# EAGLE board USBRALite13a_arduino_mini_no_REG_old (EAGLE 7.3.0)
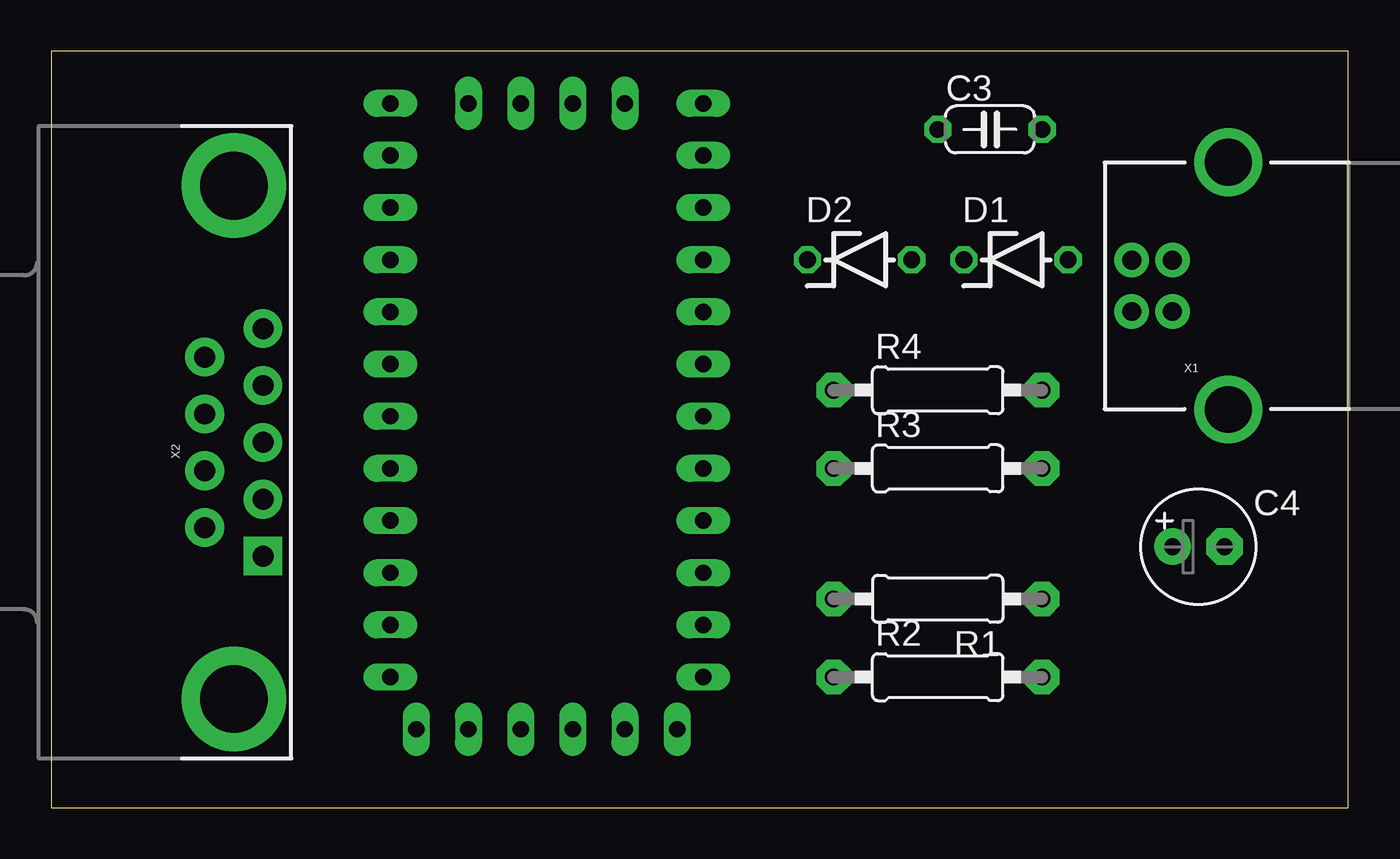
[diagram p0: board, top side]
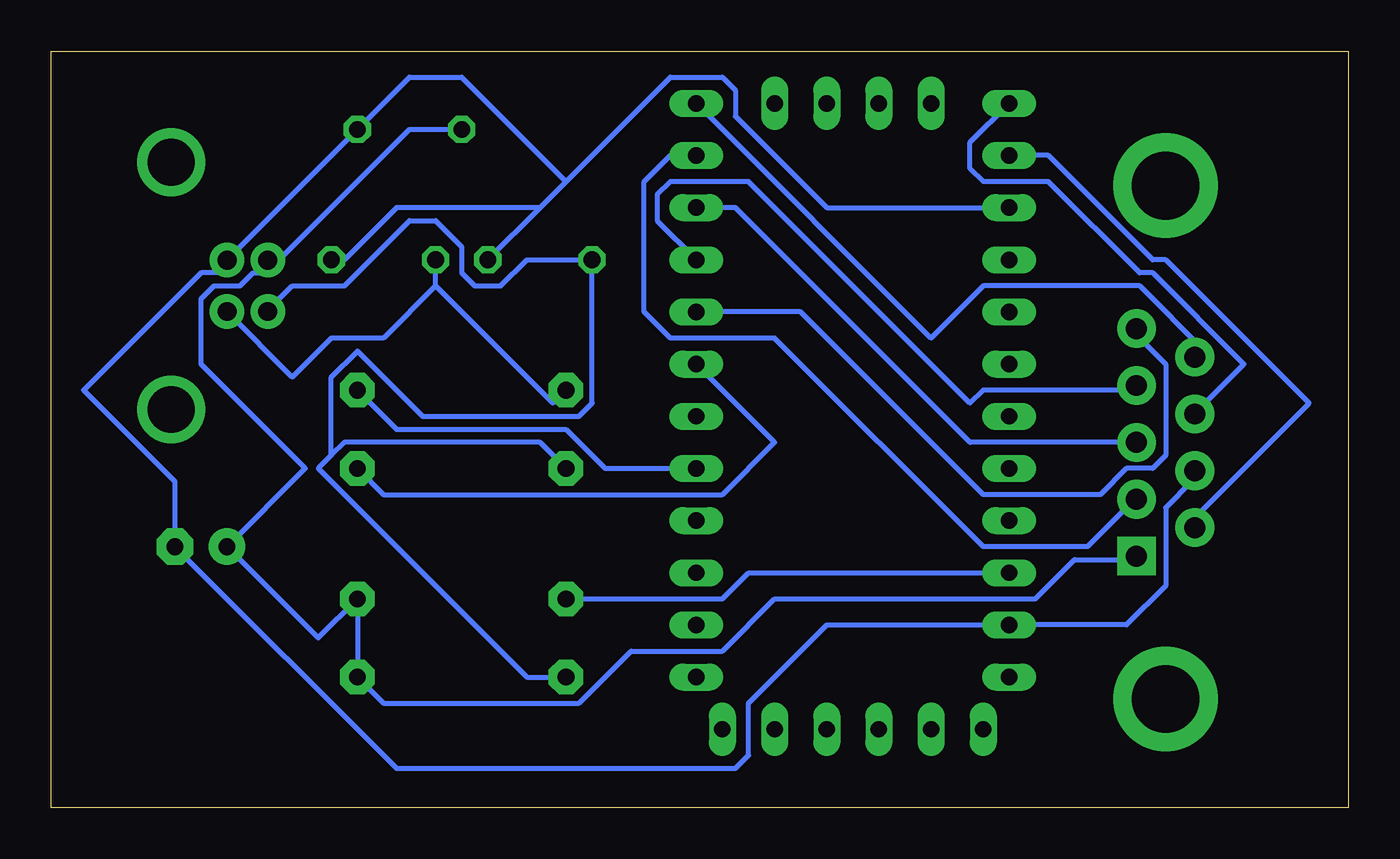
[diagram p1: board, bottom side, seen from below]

Size 63.17 x 36.82 mm. Coordinates in mm from the lower left corner, seen from the top.
Outline: 0,0 63.17,0 63.17,36.82 0,36.82 0,0
Copper layers (1*16): Top 0.035mm / dielectric 1.5mm / Bottom 0.035mm
Design rules "default": minimum track width 10mil, minimum drill 24mil, track to track 8mil, track to pad 8mil, pad to pad 8mil, via to via 8mil, smd to smd 8mil, copper to edge 40mil, drill to drill 8mil, minimum pad ring 10mil, minimum via ring 8mil, stop-mask expansion 4mil, vias tented up to drill 0mil, thermal gap 10mil

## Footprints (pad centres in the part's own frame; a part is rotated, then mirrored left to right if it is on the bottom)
C050-024X044 = drill 0.813 octagon: 1 -2.54,0; 2 2.54,0
E2,5-6 = drill 0.813 pad 1.778: + -1.27,0 | drill 0.813 pad 1.778 octagon: - 1.27,0
ZDIO-5 = drill 0.813 octagon: A 2.54,0; C -2.54,0
0207/10 = drill 0.813 pad 1.676 octagon: 1 -5.08,0; 2 5.08,0
PRO-MINI = drill 0.8 long: A0 8.89,8.89; A1 8.89,11.43; A2 8.89,13.97; A3 8.89,16.51; A4 -2.54,-1.27; A5 0,-1.27; A6 2.54,-1.27; A7 5.08,-1.27; D2 -6.35,16.51; D3 -6.35,13.97; D4 -6.35,11.43; D5 -6.35,8.89; D6 -6.35,6.35; D7 -6.35,3.81; D8 -6.35,1.27; D9 -6.35,-1.27; D10 8.89,-1.27; D11 8.89,1.27; D12 8.89,3.81; D13 8.89,6.35; DTR 7.62,29.21; GND 8.89,24.13; GND1 -6.35,19.05; GND2 -5.08,29.21; GND3 -2.54,29.21; RAW 8.89,26.67; RST 8.89,21.59; RST1 -6.35,21.59; RX1 -6.35,24.13; RX1-1 2.54,29.21; TX0 -6.35,26.67; TX0-1 5.08,29.21; VCC 8.89,19.05; VCC1 0,29.21
USB-B-PTH = drill 0.914 pad 1.676: D+ 0,1.25; D- 1.981,1.25; GND 0,-1.25; VBUS 1.981,-1.25 | drill 2.286: S1 -2.718,-6.02; S2 -2.718,6.02
DB9_MALE = drill 1.016 pad 1.88: 1 5.54,-1.42; 2 2.77,-1.42; 3 0,-1.42; 4 -2.77,-1.42; 6 4.15,1.42; 7 1.38,1.42; 8 -1.38,1.42; 9 -4.15,1.42 | drill 1.016 pad 1.88 square: 5 -5.54,-1.42 | drill 3.302 pad 5.08: G1 -12.5,0; G2 12.5,0

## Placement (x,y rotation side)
C3  0.1uF  [C050-024X044]  45.72,33.02 0 top
C4  4u7  [E2,5-6]  55.88,12.7 0 top
D1  3V6  [ZDIO-5]  46.99,26.67 0 top
D2  3V6  [ZDIO-5]  39.37,26.67 0 top
R1  10K  [0207/10]  43.18,10.16 180 top
R2  1K5  [0207/10]  43.18,6.35 0 top
R3  68R  [0207/10]  43.18,16.51 0 top
R4  68R  [0207/10]  43.18,20.32 0 top
U$1  PRO-MINI  [PRO-MINI]  25.4,33.02 180 top
X1  USBPTH  [USB-B-PTH]  54.61,25.4 180 top
X2  [DB9_MALE]  8.89,17.78 90 top

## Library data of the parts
C3 = rcl
C4 R1-R4 = adafruit
D1 D2 = diode
U$1 = Arduino-clone
X1 X2 = SparkFun

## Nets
D+: R4.2 U$1.D2
D-: R3.2 U$1.D4
GND: C3.2 C4.- D1.A D2.A U$1.D12 U$1.GND X1.GND X2.8
N$1: R1.2 U$1.RST
N$8: D1.C R4.1 X1.D+
N$9: D2.C R2.1 R3.1 X1.D-
PB0: U$1.D8 X2.4
PB1: U$1.D9 X2.6
PB2: U$1.D10 X2.7
PB3: U$1.D11 X2.9
PD5: U$1.D5 X2.1
PD7: U$1.D7 X2.3
PD62: U$1.D6 X2.2
RAW: U$1.RAW
VCC: C3.1 C4.+ R1.1 R2.2 X1.VBUS X2.5

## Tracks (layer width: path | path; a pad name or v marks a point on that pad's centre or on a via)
D+
  Bottom 0.254: U$1.D2 36.2,16.51 38.1,18.41 46.35,18.41 R4.2
D-
  Bottom 0.254: U$1.D4 27.94,17.78 30.48,15.24 46.99,15.24 R3.2
GND
  Bottom 0.254: U$1.D12 25.4,29.21 29.84,33.66 29.84,34.92 30.48,35.56 33.02,35.56 38.1,30.48 | D2.A 39.37,29.21 | 39.37,29.21 38.1,30.48 | D1.A 48.9,26.67 46.35,29.21 39.37,29.21 | X2.8 7.62,15.88 8.89,14.6 8.89,10.79 10.79,8.89 U$1.GND 25.4,8.89 29.21,5.08 29.21,2.54 29.84,1.9 46.35,1.9 C4.- 57.15,15.88 61.59,20.32 55.88,26.03 54.61,26.03 X1.GND 54.61,26.67 C3.2 45.72,35.56 43.18,35.56 38.1,30.48
N$1
  Bottom 0.254: U$1.RST 29.21,11.43 30.48,10.16 R1.2
N$8
  Bottom 0.254: 44.45,25.4 D1.C | 44.45,25.4 38.73,19.69 R4.1 | 44.45,25.4 46.99,22.86 49.53,22.86 51.44,20.95 54.61,24.13 X1.D+
N$9
  Bottom 0.254: X1.D- 52.07,24.77 51.44,25.4 48.9,25.4 45.72,28.58 44.45,28.58 43.18,27.3 43.18,26.03 42.55,25.4 41.27,25.4 40.01,26.67 D2.C 36.83,19.69 37.47,19.05 45.09,19.05 48.26,22.22 49.53,20.95 49.53,17.14 | R2.1 40.01,6.35 50.16,16.51 49.53,17.14 | 49.53,17.14 48.9,17.78 39.37,17.78 R3.1
PB0
  Bottom 0.254: U$1.D8 33.02,31.75 34.29,30.48 34.29,24.13 33.02,22.86 27.94,22.86 17.78,12.7 12.7,12.7 10.79,14.6 X2.4
PB1
  Bottom 0.254: U$1.D9 20.32,22.86 17.78,25.4 10.16,25.4 6.99,22.22 X2.6
PB2
  Bottom 0.254: U$1.D10 18.41,32.38 18.41,31.11 17.78,30.48 14.61,30.48 10.16,26.03 9.53,26.03 5.08,21.59 6.99,19.69 X2.7
PB3
  Bottom 0.254: U$1.D11 14.61,31.75 9.53,26.67 8.89,26.67 1.91,19.69 7.62,13.97 X2.9
PD5
  Bottom 0.254: U$1.D5 26.67,24.13 17.78,15.24 12.06,15.24 10.79,16.51 9.53,16.51 8.89,17.14 8.89,21.59 10.16,22.86 X2.1
PD7
  Bottom 0.254: U$1.D7 29.84,29.21 18.41,17.78 X2.3
PD62
  Bottom 0.254: U$1.D6 33.66,28.58 33.66,29.84 33.02,30.48 29.21,30.48 18.41,19.69 17.78,20.32 10.79,20.32 X2.2
VCC
  Bottom 0.254: C3.1 45.72,33.02 52.07,26.67 X1.VBUS 52.7,26.03 53.34,26.03 53.98,25.4 55.24,25.4 55.88,24.77 55.88,21.59 50.8,16.51 C4.+ 50.16,8.25 R1.1 R2.2 46.99,5.08 37.47,5.08 34.92,7.62 30.48,7.62 27.94,10.16 15.24,10.16 13.34,12.06 10.79,12.06 X2.5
